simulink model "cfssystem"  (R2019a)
settings: configuration reference "configurationSettings" (kept in a data dictionary, not in this file)

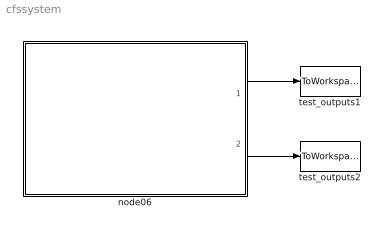
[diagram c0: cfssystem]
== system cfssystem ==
  node06 : ModelReference  ModelNameDialog=SCD_rtc_06.slx  SimulationMode=Normal  ModelReferenceVersion=1.18
  test_outputs1 : ToWorkspace  VariableName=cfs1simout  SaveFormat=Timeseries  SampleTime=-1
  test_outputs2 : ToWorkspace  VariableName=cfs2simout  SaveFormat=Timeseries  SampleTime=-1
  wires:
  node06/1 -> test_outputs1/1
  node06/2 -> test_outputs2/1
